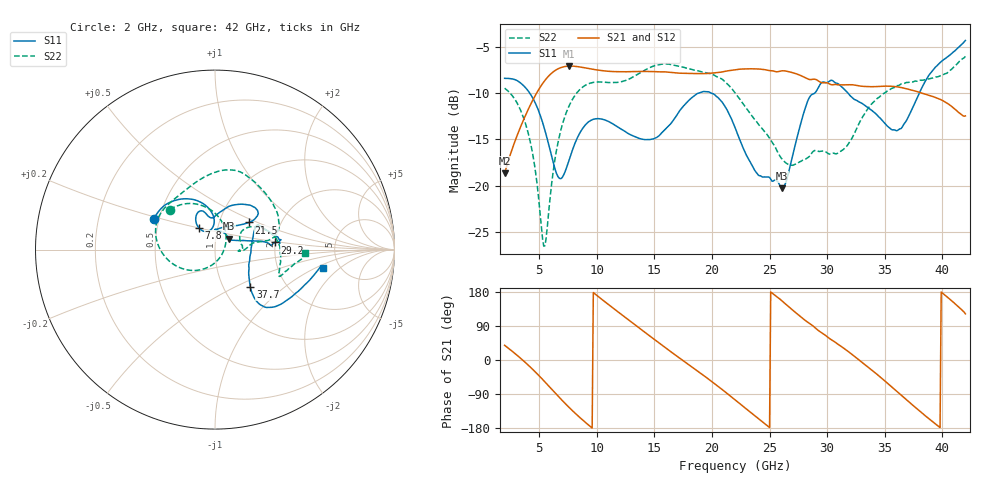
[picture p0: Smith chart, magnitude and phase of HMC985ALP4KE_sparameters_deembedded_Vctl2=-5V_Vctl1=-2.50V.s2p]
!s2p File: Measurements: S11, S21, S12, S22
# GHz S dB R 50.0
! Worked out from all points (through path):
!   401 points, 2 GHz to 42 GHz, reference 50 ohm
!   highest |S21| = -7.05 dB at 7.6 GHz (marker M1); lowest = -18.7 dB at 2 GHz (marker M2)
!   lowest |S11| = -20.3 dB at 26.1 GHz (marker M3), VSWR 1.21, Z = 57.7 + j7.02 ohm
!   |S11| at or under -10 dB: 4.191 GHz to 18.79 GHz (14.6 GHz wide, 127 % of centre); 19.97 GHz to 28.91 GHz (8.941 GHz wide, 36.6 % of centre); 31.82 GHz to 37.99 GHz (6.169 GHz wide, 17.7 % of centre)
!   |S22| runs from -26.6 to -6.0 dB; largest |S21 - S12| = 0.00047
!   S11 on the Smith chart (normalised r, x): 2 GHz: 0.47, +0.19; 7.8 GHz: 0.81, +0.20; 21.5 GHz: 1.39, +0.45; 29.2 GHz: 1.99, +0.18; 37.7 GHz: 1.33, -0.61; 42 GHz: 3.71, -1.22
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2  -8.38 153.3  -18.68 38.9  -18.69 38.9  -9.45 138.6
4  -9.67 120.4  -11.88 -12.1  -11.88 -12.1  -14.09 88.4
5.4  -13.58 95.3  -8.77 -54.6  -8.77 -54.6  -26.56 -17.6
6.7  -19.14 105.1  -7.31 -97.1  -7.32 -97.1  -14.95 -139.8
7.6  -17.22 125.8  -7.05 -125.2  -7.06 -125.2  -11.35 -168.5
7.8  -16.47 126.6  -7.06 -131.2  -7.06 -131.2  -10.86 -173.7
8.7  -13.95 122.4  -7.18 -156.4  -7.19 -156.4  -9.40 166.8
10.4  -12.79 109.7  -7.54 160.9  -7.54 160.9  -8.78 142.0
12.4  -14.09 102.9  -7.67 114.2  -7.67 114.2  -8.65 117.1
15.4  -14.61 90.0  -7.68 45.1  -7.68 45.1  -6.90 79.4
18.3  -10.43 56.8  -7.86 -19.1  -7.86 -19.1  -7.44 51.6
21.5  -12.29 38.6  -7.54 -92.7  -7.55 -92.7  -9.20 13.2
22  -13.68 42.8  -7.45 -105.1  -7.45 -105.0  -9.94 10.7
24.1  -18.92 85.8  -7.37 -156.3  -7.38 -156.2  -13.46 9.5
26.1  -20.29 38.5  -7.56 155.5  -7.57 155.5  -17.15 -3.5
28.7  -10.11 4.2  -8.50 91.5  -8.50 91.6  -16.41 3.3
29.2  -9.46 6.8  -8.63 78.7  -8.64 78.7  -16.27 3.8
32.4  -10.69 24.8  -9.11 8.9  -9.11 8.9  -14.25 35.0
35.4  -13.73 6.6  -9.23 -65.6  -9.23 -65.5  -9.65 14.9
37.7  -10.82 -46.8  -9.78 -126.3  -9.78 -126.2  -8.67 -6.1
39.7  -6.79 -44.3  -10.59 -176.0  -10.59 -175.9  -8.16 -22.5
42  -4.28 -9.7  -12.45 121.7  -12.46 121.8  -6.00 -2.4
